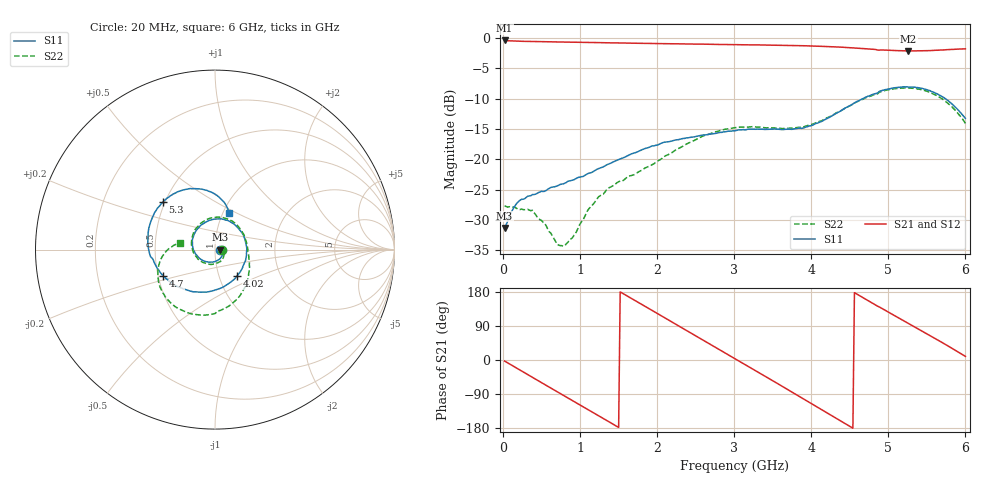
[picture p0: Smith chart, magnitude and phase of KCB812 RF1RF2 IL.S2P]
!Agilent Technologies,E5071B,JP1KK00126,A.08.11
!Date: Tue May 14 08:32:30 2013
!Data & Calibration Information:
!Freq	S11:SOLT2(ON)	S21:SOLT2(ON)	S12:SOLT2(ON)	S22:SOLT2(ON)
# Hz S dB R 50
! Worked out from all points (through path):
!   300 points, 20 MHz to 6 GHz, reference 50 ohm
!   highest |S21| = -0.44 dB at 20 MHz (marker M1); lowest = -2.2 dB at 5.26 GHz (marker M2)
!   group delay of S21, straight-line fit = 329 ps
!   lowest |S11| = -31.3 dB at 20 MHz (marker M3), VSWR 1.06, Z = 52.8 + j0.0174 ohm
!   |S11| at or under -10 dB: start of sweep to 4.672 GHz; 5.738 GHz to end of sweep
!   |S22| runs from -34.3 to -8.2 dB; largest |S21 - S12| = 0.0039
!   S11 on the Smith chart (normalised r, x): 20 MHz: 1.06, +0.00; 4.02 GHz: 1.22, -0.37; 4.7 GHz: 0.53, -0.18; 5.3 GHz: 0.49, +0.30; 6 GHz: 1.08, +0.46
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2e7  -31.30 0.3  -0.44 -2.8  -0.43 -2.9  -27.68 0.7
2e8  -26.98 -10.6  -0.56 -24.3  -0.55 -24.4  -28.28 -7.8
5.6e8  -25.13 -54.7  -0.64 -66.9  -0.64 -67.0  -30.97 -32.7
7.8e8  -24.06 -80.7  -0.70 -93.0  -0.70 -93.1  -34.32 -15.3
1.02e9  -22.87 -105.2  -0.75 -121.3  -0.74 -121.3  -30.26 1.7
1.28e9  -21.36 -130.1  -0.80 -152.0  -0.79 -152.0  -25.83 -17.7
1.52e9  -19.96 -153.6  -0.84 179.7  -0.84 179.6  -23.62 -48.7
1.76e9  -18.68 -175.5  -0.90 151.3  -0.89 151.3  -22.07 -87.7
2.02e9  -17.57 162.4  -0.95 120.7  -0.95 120.6  -20.19 -133.1
2.48e9  -16.33 125.8  -1.03 66.4  -1.02 66.3  -16.91 153.9
2.78e9  -15.68 103.4  -1.09 30.9  -1.08 30.7  -15.42 112.5
3.02e9  -15.28 82.4  -1.12 2.5  -1.12 2.3  -14.79 83.0
3.28e9  -15.06 56.5  -1.17 -28.5  -1.17 -28.5  -14.69 53.8
3.56e9  -15.04 22.1  -1.23 -61.9  -1.21 -62.0  -14.87 24.9
4.02e9  -14.37 -49.8  -1.35 -117.3  -1.35 -117.3  -14.19 -14.3
4.36e9  -12.21 -105.3  -1.52 -158.3  -1.51 -158.3  -12.16 -42.6
4.7e9  -9.81 -152.6  -1.80 161.1  -1.79 161.2  -9.91 -73.9
5.02e9  -8.40 168.8  -2.06 124.1  -2.05 124.2  -8.53 -104.0
5.26e9  -8.11 142.1  -2.16 96.7  -2.15 96.8  -8.25 -127.0
5.3e9  -8.09 137.8  -2.16 92.2  -2.17 92.2  -8.29 -130.8
5.64e9  -9.27 102.0  -2.05 53.0  -2.05 53.1  -9.62 -162.7
6e9  -13.26 68.3  -1.82 9.6  -1.82 9.7  -14.09 169.2
